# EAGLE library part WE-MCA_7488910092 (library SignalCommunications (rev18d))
Multilayer Chip Antenna Characteristics SMD Multilayer Chip Antenna Extremely low profile Very light component Power capacity: 5 W max. Omni-directional Operating temperature: –40 °C to +85 °C High gain Applications applications WLAN Home RF (868 MHz) Bluetooth applications GSM 900 ISM 868/2400 Details see: http://katalog.we-online.de/en/pbs/WE-MCA? Updated by Dan Xu 2014-07-08 2014 (C) Wurth Elektronik
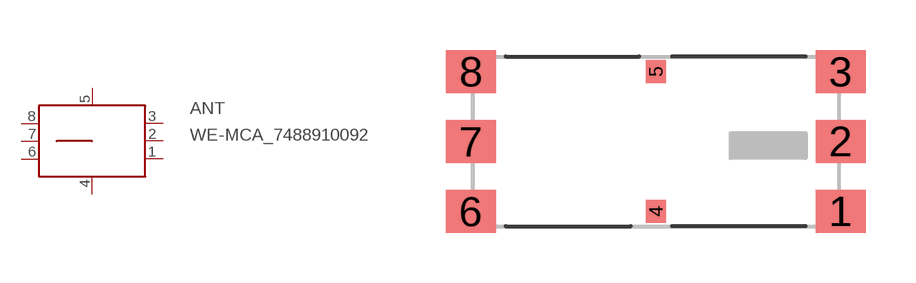
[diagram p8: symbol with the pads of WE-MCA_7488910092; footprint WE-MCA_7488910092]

Designator prefix ANT

## WE-MCA_7488910092  [WE-MCA_7488910092]
1  NC1  nc
2  FD  nc
3  NC2  nc
4  NC3  nc
5  NC4  nc
6  NC5  nc
7  NC6  pas
8  NC7  nc

## Footprint WE-MCA_7488910092 (pad centres in mm)
Multilayer Chip Antenna WE-MCA
smd 1.5 x 1.3: 1 5.55,-2.1; 2 5.55,0; 3 5.55,2.1; 6 -5.55,-2.1; 7 -5.55,0; 8 -5.55,2.1
smd 0.6 x 0.7: 4 0,-2.1; 5 0,2.1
